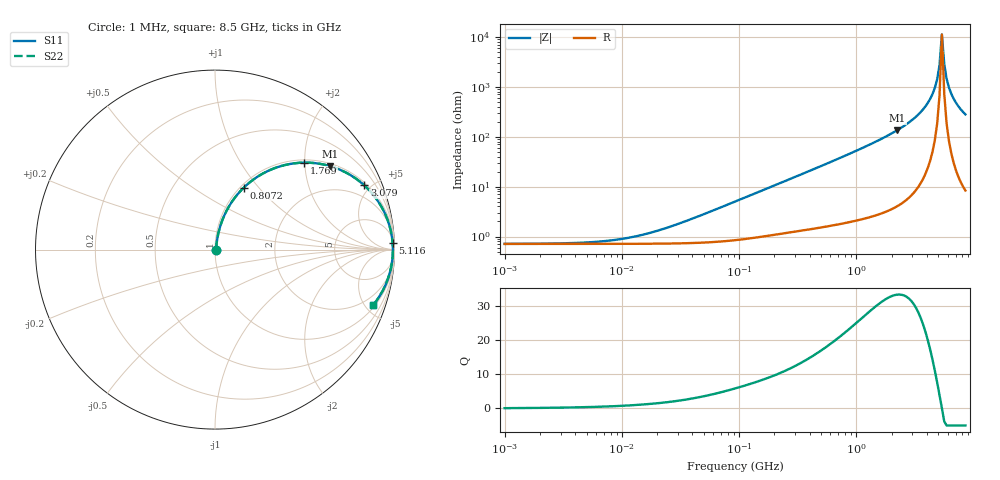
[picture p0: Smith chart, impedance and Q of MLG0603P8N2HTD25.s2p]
! S-Parameter Data Generated by TDK Corporation
! Copyright(C) 2025 TDK Corporation.
! All Rights Reserved.
! TDK P/N: MLG0603P8N2HTD25 (SMD / SMT Inductor (Coil))
! Property: L=8.2nH at 500MHz
! Size(LxWxT): 0.6x0.3x0.3mm
! Model Type: s2p (Touchstone File Format Version 1.0)
! Frequency: DC=Yes Start=1MHz Stop=8500MHz 198points Log-sweep
! Model Generated on Feb. 6, 2025
! Terms and conditions regarding TDK Simulation Models:
! 1)This simulation model is being provided solely for informational
!  purposes. Please refer to the specifications of the products in
!  terms of detailed characteristics of such products.
! 2)In no event shall TDK Corporation of any of its subsidiaries be
!  liable for any loss or damage arising, directly or indirectly,
!  from any information contained in this simulation model, including,
!  but not limited to loss or damages arising from any inaccuracies,
!  omissions or errors in connection with such information.
! 3)Any and all copyrights on this simulation model are owned by
!  TDK Corporation.  Duplication or redistribution of this simulation
!  model without prior written permission from TDK Corporation
!  is prohibited.
! 4)This simulation model is subject to any modification or change
!  without any prior notice.
! 5)Neither TDK Corporation nor any of its subsidiaries shall make any
!  warranty, express or implied, including but not limited to the
!  correctness, implied warranties of merchantability and fitness for
!  a particular purpose with respect to this simulation models.
! 6)The use of this simulation model shall be deemed to have consented
!  to the terms and conditions hereof.
! Port Assignments:
!  1 ---@@@--- 2
! Applicable Conditions:
!  Temperature = 25 degC
!  DC Bias Current = 0 A
!  Small Signal Operation
# Hz S MA R 50
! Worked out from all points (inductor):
!   197 points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, 1 MHz to 8.5 GHz, reference 50 ohm
!   read as one part in series: L = 8.58 nH near 42.06 MHz
!   highest Q = 33.4 at 2.229 GHz (marker M1), where L = 9.62 nH
!   self-resonance near 5.357 GHz
!   S11 on the Smith chart (normalised r, x): 1 MHz: 1.01, +0.00; 807.2 MHz: 1.04, +0.84; 1.769 GHz: 1.06, +1.99; 3.079 GHz: 1.15, +4.58; 5.116 GHz: 14, +53; 8.5 GHz: 1.17, -5.59
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1000000  0.007071 4.3  0.9929 -0.0  0.9929 -0.0  0.007071 4.3
4587603  0.007473 19.1  0.9929 -0.1  0.9929 -0.1  0.007473 19.1
1.005548e7  0.008901 37.1  0.9929 -0.3  0.9929 -0.3  0.008901 37.1
2.10461e7  0.01337 57.1  0.9928 -0.6  0.9928 -0.6  0.01337 57.1
9.219544e7  0.04956 77.5  0.9905 -2.8  0.9905 -2.8  0.04956 77.5
4.229561e8  0.2108 74.1  0.9639 -12.1  0.9639 -12.1  0.2108 74.1
8.071757e8  0.3801 65.1  0.9081 -22.3  0.9081 -22.3  0.3801 65.1
1.769233e9  0.6947 44.2  0.698 -44.0  0.698 -44.0  0.6947 44.2
1.940355e9  0.7344 41.0  0.6567 -47.2  0.6567 -47.2  0.7344 41.0
2.228565e9  0.7917 36.0  0.5876 -52.3  0.5876 -52.3  0.7917 36.0
3.07866e9  0.9057 23.3  0.3954 -64.9  0.3954 -64.9  0.9057 23.3
3.703002e9  0.952 15.7  0.2701 -72.0  0.2701 -72.0  0.952 15.7
4.253027e9  0.9754 9.8  0.1712 -76.9  0.1712 -76.9  0.9754 9.8
4.664383e9  0.9853 5.9  0.1038 -78.9  0.1038 -78.9  0.9853 5.9
4.884749e9  0.9885 4.0  0.06997 -78.5  0.06997 -78.5  0.9885 4.0
5.115526e9  0.9904 2.0  0.03632 -73.7  0.03632 -73.7  0.9904 2.0
5.357206e9  0.9912 0.1  0.008884 -6.1  0.008884 -6.1  0.9912 0.1
5.610304e9  0.9907 -1.9  0.03444 73.4  0.03444 73.4  0.9907 -1.9
5.87536e9  0.989 -3.9  0.0681 78.8  0.0681 78.8  0.989 -3.9
6.152938e9  0.9861 -5.8  0.1021 79.3  0.1021 79.3  0.9861 -5.8
7.066863e9  0.9702 -11.7  0.2032 75.8  0.2032 75.8  0.9702 -11.7
8.5e9  0.9328 -19.5  0.3336 68.8  0.3336 68.8  0.9328 -19.5
